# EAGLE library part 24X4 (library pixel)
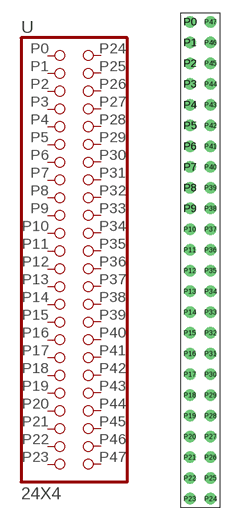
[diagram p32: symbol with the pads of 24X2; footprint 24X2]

Designator prefix -

## 24X4  [24X2]
P0  P0  pas
P1  P1  pas
P2  P2  pas
P3  P3  pas
P4  P4  pas
P5  P5  pas
P6  P6  pas
P7  P7  pas
P8  P8  pas
P9  P9  pas
P10  P10  pas
P11  P11  pas
P12  P12  pas
P13  P13  pas
P14  P14  pas
P15  P15  pas
P16  P16  pas
P17  P17  pas
P18  P18  pas
P19  P19  pas
P20  P20  pas
P21  P21  pas
P22  P22  pas
P23  P23  pas
P24  P24  pas
P25  P25  pas
P26  P26  pas
P27  P27  pas
P28  P28  pas
P29  P29  pas
P30  P30  pas
P31  P31  pas
P32  P32  pas
P33  P33  pas
P34  P34  pas
P35  P35  pas
P36  P36  pas
P37  P37  pas
P38  P38  pas
P39  P39  pas
P40  P40  pas
P41  P41  pas
P42  P42  pas
P43  P43  pas
P44  P44  pas
P45  P45  pas
P46  P46  pas
P47  P47  pas

## Footprint 24X2 (pad centres in mm)
drill 0.9 pad 1.27: P0 -1.27,29.21; P1 -1.27,26.67; P2 -1.27,24.13; P3 -1.27,21.59; P4 -1.27,19.05; P5 -1.27,16.51; P6 -1.27,13.97; P7 -1.27,11.43; P8 -1.27,8.89; P9 -1.27,6.35; P10 -1.27,3.81; P11 -1.27,1.27; P12 -1.27,-1.27; P13 -1.27,-3.81; P14 -1.27,-6.35; P15 -1.27,-8.89; P16 -1.27,-11.43; P17 -1.27,-13.97; P18 -1.27,-16.51; P19 -1.27,-19.05; P20 -1.27,-21.59; P21 -1.27,-24.13; P22 -1.27,-26.67; P23 -1.27,-29.21; P24 1.27,-29.21; P25 1.27,-26.67; P26 1.27,-24.13; P27 1.27,-21.59; P28 1.27,-19.05; P29 1.27,-16.51; P30 1.27,-13.97; P31 1.27,-11.43; P32 1.27,-8.89; P33 1.27,-6.35; P34 1.27,-3.81; P35 1.27,-1.27; P36 1.27,1.27; P37 1.27,3.81; P38 1.27,6.35; P39 1.27,8.89; P40 1.27,11.43; P41 1.27,13.97; P42 1.27,16.51; P43 1.27,19.05; P44 1.27,21.59; P45 1.27,24.13; P46 1.27,26.67; P47 1.27,29.21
